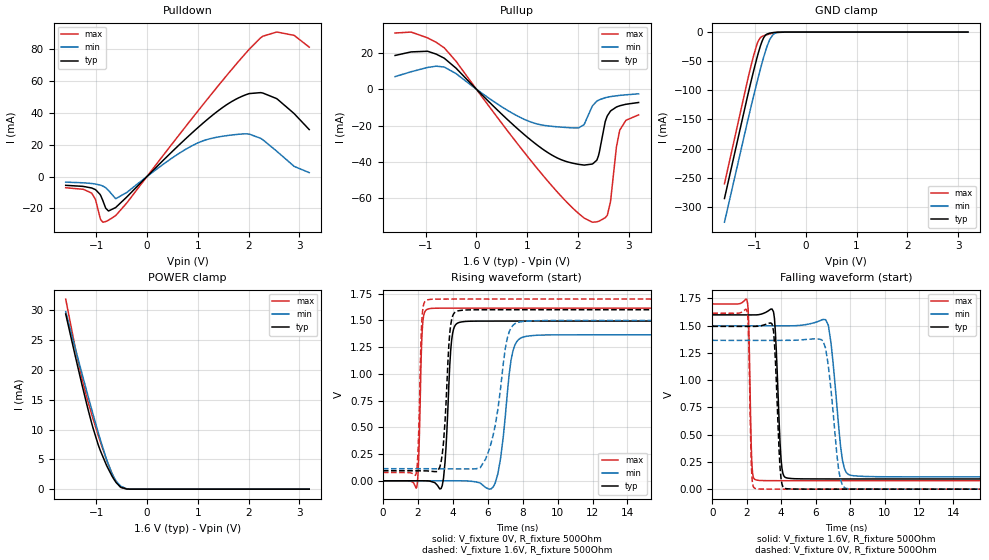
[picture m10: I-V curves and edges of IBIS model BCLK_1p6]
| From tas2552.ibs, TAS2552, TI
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|   Model
[Model]   BCLK_1p6
Model_type   I/O
Polarity   Non-Inverting
Enable   Active-Low
Vinl = 0.48
Vinh = 1.12
Vmeas = 0.8
Vref = 0
Cref = 1pF
Rref = 1000000
|   typ   min   max
C_comp   1.269pF   1.168pF   1.417pF
[Voltage Range]   1.6   1.5   1.7
[Temperature Range]   27   125   -40
[Pullup Reference]   1.6   1.5   1.7
[Pulldown Reference]   -0   -0   -0
[Power Clamp Reference]   1.6   1.5   1.7
[GND Clamp Reference]   -0   -0   -0
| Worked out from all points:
|   slope of the pulldown table from 0 to 0.24 V, typ, clamps not added: 31.3 ohm
|   slope of the pullup table from 0 to 0.24 V, typ, clamps not added: 35.7 ohm
|   GND clamp passes 1 mA (typ) near -0.65 V on its own axis
|   POWER clamp passes 1 mA (typ) near -0.59 V on its own axis
|   falling waveform, V_fixture 1.6V, R_fixture 500Ohm: 20-80 % time 237ps typ, 479ps min, 125ps max; typ from 1.6 V to 0.094 V
|   rising waveform, V_fixture 0V, R_fixture 500Ohm: 20-80 % time 264ps typ, 520ps min, 148ps max; typ from 0 V to 1.49 V
|   rising waveform, V_fixture 1.6V, R_fixture 500Ohm: 20-80 % time 303ps typ, 738ps min, 156ps max; typ from 0.094 V to 1.6 V
|   falling waveform, V_fixture 0V, R_fixture 500Ohm: 20-80 % time 238ps typ, 502ps min, 124ps max; typ from 1.49 V to 0 V
[Pulldown]
|   Voltage   I(typ)   I(min)   I(max)
-1.6V     -5.533mA   -3.513mA   -7.061mA
-1.091V   -7.185mA   -4.372mA   -10.37mA
-1.01V    -8.343mA   -4.731mA   -14.92mA
-908.8mV  -12.08mA   -5.499mA   -27.24mA
-755.2mV  -21.65mA   -8.809mA   -27.43mA
-611.2mV  -19.34mA   -13.87mA   -24.39mA
944mV     29.06mA    20.27mA    38.81mA
1.909V    50.95mA    26.81mA    76.26mA
2.245V    52.74mA    23.92mA    87.41mA
2.547V    49.08mA    16.16mA    90.8mA
2.893V    39.74mA    6.541mA    88.81mA
3.195V    29.53mA    2.453mA    81.37mA
[GND Clamp]
|   Voltage   I(typ)   I(min)   I(max)
-1.6V     -285.8mA   -326.4mA   -260.4mA
-1.144V   -109.4mA   -152.7mA   -82.22mA
-1.024V   -65.93mA   -109mA     -39.78mA
-961.6mV  -44.78mA   -86.98mA   -21.39mA
-899.2mV  -25.78mA   -65.76mA   -10.18mA
-860.8mV  -16.07mA   -53.27mA   -7.551mA
-812.8mV  -7.549mA   -38.56mA   -5.873mA
-707.2mV  -1.776mA   -12.66mA   -3.149mA
-635.2mV  -760.5uA   -3.656mA   -1.651mA
-558.4mV  -217.6uA   -695.8uA   -559.3uA
-400mV    -4.94uA    -14.22uA   -10.78uA
3.195V    0A         0A         0A
[Pullup]
|   Voltage   I(typ)   I(min)   I(max)
-1.6V     18.53mA    6.89mA     30.87mA
-961.6mV  20.83mA    11.92mA    28.22mA
-630.4mV  16.98mA    12.14mA    22.7mA
1.213V    -31.07mA   -19.26mA   -44.1mA
2.014V    -41.36mA   -21.3mA    -68.4mA
2.278V    -41.22mA   -9.612mA   -73.12mA
2.403V    -36.77mA   -6.12mA    -72.71mA
2.538V    -17.87mA   -4.713mA   -70.73mA
2.638V    -12.19mA   -4.134mA   -62.33mA
2.758V    -9.831mA   -3.655mA   -31.85mA
2.821V    -9.176mA   -3.455mA   -22.9mA
3.195V    -7.34mA    -2.576mA   -14.14mA
[POWER Clamp]
|   Voltage   I(typ)   I(min)   I(max)
-1.6V     29.37mA    29.76mA    31.88mA
-1.418V   22.54mA    23.82mA    23.92mA
-1.283V   17.65mA    19.5mA     18.67mA
-1.086V   11mA       13.31mA    12.5mA
-966.4mV  7.615mA    9.697mA    9.202mA
-803.2mV  4.135mA    5.186mA    5.107mA
-692.8mV  2.269mA    2.718mA    2.722mA
-601.6mV  1.06mA     1.301mA    1.173mA
-524.8mV  391.5uA    565.6uA    362.6uA
-400mV    29.86uA    73.87uA    17.64uA
-289.6mV  1.33uA     6.493uA    403.9nA
3.195V    0A         0A         0A
[Ramp]
R_load = 500
|   typ   min   max
dV/dt_r   0.896442/2.63657e-10   0.819506/5.20383e-10   0.968975/1.47751e-10
dV/dt_f   0.903756/2.36927e-10   0.832139/4.78618e-10   0.973375/1.24815e-10
[Falling Waveform]
V_fixture = 1.6V
V_fixture_min = 1.5V
V_fixture_max = 1.7V
R_fixture = 500Ohm
C_fixture = 0F
|   Time   V(typ)   V(min)   V(max)
0s        1.6V       1.5V       1.7V
2.011ns   1.599V     1.5V       1.737V
2.315ns   1.599V     1.5V       194.7mV
2.705ns   1.602V     1.5V       80.41mV
3.556ns   1.627V     1.499V     77.95mV
4.045ns   191.7mV    1.499V     77.77mV
4.576ns   97.92mV    1.5V       77.71mV
6.737ns   93.78mV    1.506V     77.71mV
8.264ns   93.76mV    122.3mV    77.71mV
100ns     93.74mV    113.1mV    77.71mV
[Rising Waveform]
V_fixture = 0V
V_fixture_min = 0V
V_fixture_max = 0V
R_fixture = 500Ohm
C_fixture = 0F
|   Time   V(typ)   V(min)   V(max)
0s        2.191nV    34nV       1.175nV
1.941ns   210.1uV    158.2uV    -56.77mV
2.266ns   245.2uV    184.7uV    1.445V
2.772ns   -7.592mV   225.9uV    1.613V
3.398ns   -44.13mV   276.9uV    1.615V
4.699ns   1.49V      -753uV     1.615V
6.427ns   1.494V     -21.62mV   1.615V
7.445ns   1.494V     1.217V     1.615V
8.662ns   1.494V     1.36V      1.615V
100ns     1.494V     1.366V     1.615V
[Rising Waveform]
V_fixture = 1.6V
V_fixture_min = 1.5V
V_fixture_max = 1.7V
R_fixture = 500Ohm
C_fixture = 0F
|   Time   V(typ)   V(min)   V(max)
0s        93.74mV    113.1mV    77.71mV
1.906ns   93.38mV    112.9mV    65.57mV
2.241ns   93.11mV    112.9mV    1.532V
2.705ns   89.81mV    112.7mV    1.697V
3.398ns   247.6mV    112mV      1.7V
3.937ns   1.51V      111.4mV    1.7V
4.576ns   1.596V     110.7mV    1.7V
5.88ns    1.6V       203.7mV    1.7V
8.131ns   1.6V       1.492V     1.7V
100ns     1.6V       1.5V       1.7V
[Falling Waveform]
|Gnd
V_fixture = 0V
V_fixture_min = 0V
V_fixture_max = 0V
R_fixture = 500Ohm
C_fixture = 0F
|   Time   V(typ)   V(min)   V(max)
0s        1.494V     1.366V     1.615V
2.011ns   1.494V     1.366V     1.638V
2.29ns    1.494V     1.366V     143.3mV
2.638ns   1.495V     1.366V     2.687mV
3.556ns   1.452V     1.366V     198.7uV
3.937ns   191.9mV    1.366V     53.73uV
4.317ns   4.432mV    1.366V     5.803uV
6.427ns   27.23uV    1.362V     5.675uV
7.887ns   17.56uV    3.804mV    5.586uV
100ns     8.421nV    43.35nV    7.488nV
